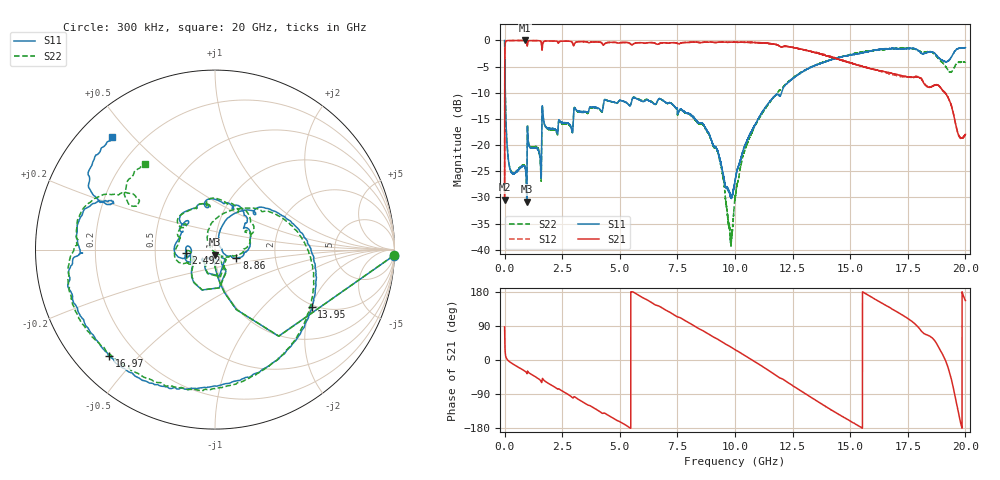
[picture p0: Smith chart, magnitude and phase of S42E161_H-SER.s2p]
! Created Wed Nov 25 22:01:58 2020
# khz S ma R 50
! 2 Port Network Data from SP1.SP block
! freq  magS11  angS11  magS21  angS21  magS12  angS12  magS22  angS22
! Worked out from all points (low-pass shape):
!   20001 points, 300 kHz to 20 GHz, reference 50 ohm
!   highest |S21| = -0.02 dB at 899.3 MHz (marker M1); lowest = -30.4 dB at 300 kHz (marker M2)
!   |S21| within 3 dB of the highest: 9.993 MHz to 14.04 GHz (14.03 GHz wide, 200 % of centre)
!   lowest |S11| = -30.8 dB at 962.3 MHz (marker M3), VSWR 1.06, Z = 50.1 - j2.89 ohm
!   |S11| at or under -10 dB: 29.94 MHz to 12.02 GHz (11.99 GHz wide, 199 % of centre)
!   |S22| runs from -39.3 to 0.0 dB; largest |S21 - S12| = 0.018
!   S11 on the Smith chart (normalised r, x): 300 kHz: 7, -57; 2.492 GHz: 0.72, -0.02; 8.86 GHz: 1.27, -0.13; 13.95 GHz: 1.92, -2.03; 16.97 GHz: 0.10, -0.41; 20 GHz: 0.10, +0.44
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300  0.9959 -2.0  0.03007 87.3  0.03015 87.9  0.9955 -1.9
109300  0.09797 -89.4  0.9937 1.5  0.9933 1.5  0.09858 -89.4
304300  0.05452 -100.1  0.9969 -8.3  0.9972 -8.4  0.055 -99.5
899300  0.05956 -122.8  0.9979 -30.2  0.9974 -30.2  0.06053 -118.0
962300  0.0289 -86.3  0.9787 -34.7  0.9778 -34.7  0.03268 -80.6
2492300  0.1644 -174.3  0.9819 -81.4  0.9825 -81.4  0.1606 -168.0
3334300  0.2085 157.3  0.9733 -108.6  0.9715 -108.6  0.2052 166.0
5175300  0.2609 102.7  0.9549 -168.7  0.9547 -168.8  0.2612 102.1
6667300  0.2733 65.0  0.9208 143.0  0.9194 143.0  0.2732 57.3
8860300  0.1292 -22.1  0.9602 68.2  0.9617 68.2  0.127 -14.2
9346300  0.0727 -27.7  0.9624 51.2  0.9639 51.2  0.06935 -35.5
9789300  0.03374 18.4  0.9603 35.3  0.9623 35.3  0.0141 -95.8
1.00003e7  0.04514 62.9  0.9616 27.4  0.9627 27.4  0.03055 152.4
1.13453e7  0.233 60.7  0.9403 -23.1  0.9384 -23.2  0.2276 70.2
1.33343e7  0.5557 -6.9  0.7767 -99.8  0.7817 -99.5  0.5593 -12.4
1.39503e7  0.6272 -30.8  0.7124 -123.2  0.7235 -123.3  0.6291 -35.0
1.54863e7  0.7575 -88.0  0.5695 -178.3  0.5676 -179.4  0.7715 -89.3
1.66673e7  0.8314 -124.2  0.4954 140.2  0.4821 140.6  0.8249 -132.9
1.69713e7  0.837 -134.7  0.4735 129.1  0.4638 129.9  0.8376 -143.8
1.89423e7  0.6538 155.7  0.3486 22.0  0.3467 22.1  0.63 150.8
1.94363e7  0.7204 156.4  0.2191 -62.6  0.2203 -62.8  0.5152 151.9
2e7  0.8511 132.0  0.1264 157.0  0.1263 158.0  0.6199 128.8
